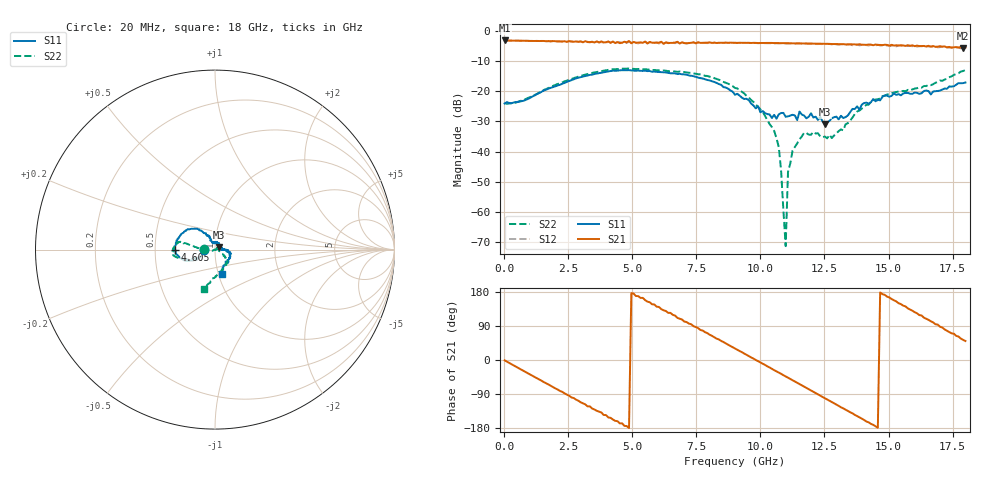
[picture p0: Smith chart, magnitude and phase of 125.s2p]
!Agilent Technologies,N5230A,US43500223,A.07.50.48
!Agilent N5230A: A.07.50.48
!Date: Wednesday, January 13, 2016 18:22:50
!Correction: S11(Full 2 Port(1,2))
!S21(Full 2 Port(1,2))
!S12(Full 2 Port(1,2))
!S22(Full 2 Port(1,2))
!S2P File: Measurements: S11, S21, S12, S22:
# Hz S  dB  R 50
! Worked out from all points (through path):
!   201 points, 20 MHz to 18 GHz, reference 50 ohm
!   highest |S21| = -3.10 dB at 20 MHz (marker M1); lowest = -5.7 dB at 17.91 GHz (marker M2)
!   group delay of S21, straight-line fit = 103 ps
!   lowest |S11| = -30.9 dB at 12.52 GHz (marker M3), VSWR 1.06, Z = 52.4 + j1.61 ohm
!   |S11| at or under -10 dB: start of sweep to end of sweep
!   |S22| runs from -71.5 to -12.4 dB; largest |S21 - S12| = 0.06
!   S11 on the Smith chart (normalised r, x): 20 MHz: 0.88, +0.00; 4.605 GHz: 0.63, -0.00; 18 GHz: 1.05, -0.29
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2e7  -24.04 179.8  -3.10 -0.9  -3.11 -0.9  -23.87 179.2
1.7281e9  -19.11 -150.8  -3.32 -64.4  -3.30 -65.3  -18.92 -155.3
3.0766e9  -15.10 -159.6  -3.71 -114.2  -3.64 -115.0  -14.67 -162.9
4.6049e9  -12.98 -179.7  -3.84 -167.1  -3.93 -170.1  -12.49 -174.6
6.0433e9  -13.59 157.9  -3.85 140.0  -4.12 138.3  -13.02 174.0
7.5716e9  -15.43 136.9  -3.73 84.1  -3.70 82.3  -14.33 167.5
9.01e9  -21.14 120.1  -3.86 30.5  -3.90 28.6  -18.91 172.5
1.05383e10  -27.84 100.4  -3.97 -26.8  -4.05 -28.5  -33.15 -165.4
1.07181e10  -27.64 95.5  -4.00 -33.3  -4.05 -35.7  -38.51 -156.5
1.0808e10  -27.21 96.5  -3.99 -36.4  -4.04 -38.4  -46.22 -171.2
1.09878e10  -28.46 96.0  -4.01 -43.4  -4.09 -45.9  -71.46 64.4
1.10777e10  -28.33 92.5  -4.00 -46.7  -4.12 -48.9  -46.83 -5.1
1.12575e10  -27.80 77.9  -4.04 -53.5  -4.11 -56.2  -39.66 21.7
1.1707e10  -28.04 63.4  -4.13 -70.4  -4.18 -72.0  -33.75 40.3
1.20666e10  -28.71 44.5  -4.16 -83.9  -4.16 -86.2  -33.48 39.8
1.25161e10  -30.95 32.7  -4.21 -100.9  -4.35 -103.0  -35.02 18.4
1.32353e10  -28.89 9.4  -4.33 -127.6  -4.42 -130.9  -32.98 -13.0
1.37747e10  -24.99 -1.2  -4.52 -148.0  -4.41 -151.6  -26.72 -31.3
1.50333e10  -21.82 -11.1  -4.81 165.1  -4.95 160.8  -20.99 -42.9
1.65616e10  -19.94 -49.9  -4.88 105.9  -5.11 102.6  -17.85 -75.4
1.79101e10  -17.28 -74.4  -5.68 53.1  -5.55 50.3  -13.26 -105.1
1.8e10  -17.08 -72.8  -5.47 50.2  -5.72 46.3  -12.94 -105.6
